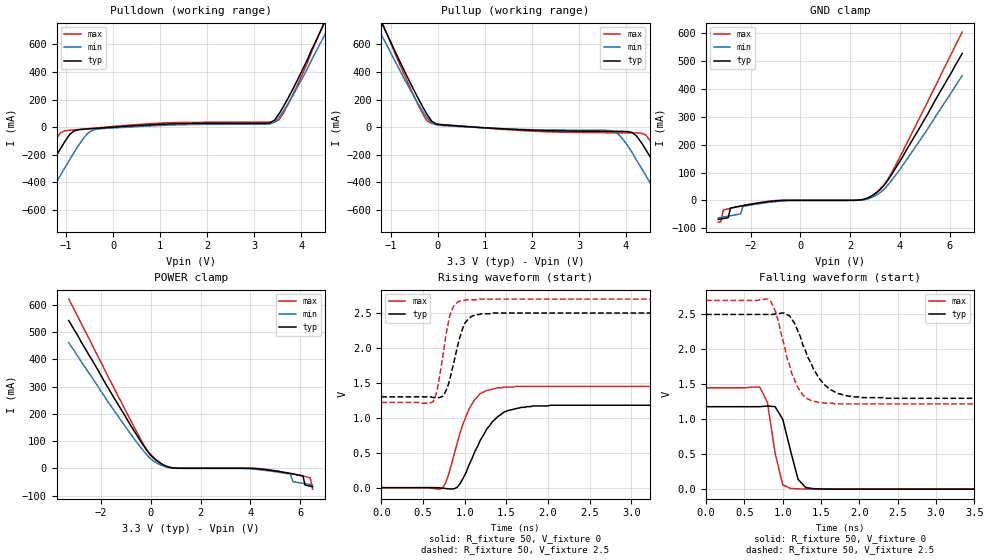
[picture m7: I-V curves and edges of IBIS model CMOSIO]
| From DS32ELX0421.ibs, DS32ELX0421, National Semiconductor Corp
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|   Model CMOSIO
[Model]  CMOSIO
Model_type I/O
Enable   Active-High
Vinl =   0
Vinh =   2
Vmeas =  1
C_comp   71.84fF   68.08fF   75.60fF
[Temperature Range]   25.0000   85.0000   -40.0000
[Voltage Range]   3.3000V   3.0000V   3.4650V
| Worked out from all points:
|   slope of the pulldown table from 0 to 0.495 V, typ, clamps not added: 44.3 ohm
|   slope of the pullup table from 0 to 0.495 V, typ, clamps not added: 36.2 ohm
|   GND clamp passes 1 mA (typ) near -0.87 V on its own axis
|   rising waveform, R_fixture 50, V_fixture 0: 20-80 % time 310ps typ, NA min, 238ps max; typ from 0 V to 1.18 V
|   rising waveform, R_fixture 50, V_fixture 2.5: 20-80 % time 151ps typ, NA min, 123ps max; typ from 1.3 V to 2.5 V
|   falling waveform, R_fixture 50, V_fixture 0: 20-80 % time 164ps typ, NA min, 139ps max; typ from 1.18 V to 0 V
|   falling waveform, R_fixture 50, V_fixture 2.5: 20-80 % time 312ps typ, NA min, 231ps max; typ from 2.5 V to 1.3 V
[GND_clamp]
|Voltage   I(typ)   I(min)   I(max)
-3.3V     -68.7mA    -62.7mA    -78.5mA
-3.2V     -67.1mA    -61.3mA    -76.7mA
-3.1V     -65.4mA    -59.8mA    -34.7mA
-2.9V     -62mA      -56.8mA    -30.4mA
-2.81V    -27.9mA    -55.3mA    -28.4mA
-2.41V    -20.8mA    -49.1mA    -20.8mA
-2.31V    -19.1mA    -21.5mA    -19mA
-1.82V    -11.5mA    -14.1mA    -10.5mA
2.44V     2.08mA     1.33mA     986uA
2.94V     20.3mA     13.6mA     19.9mA
3.73V     102mA      79.3mA     110mA
6.5V      528mA      448mA      605mA
|6.60E+00   5.43E-01   4.62E-01   6.22E-01
[POWER_clamp]
|Voltage   I(typ)   I(min)   I(max)
|6.60E+00   -6.87E-02   -6.27E-02   -7.85E-02
-3.3V     543mA      462mA      622mA
-330mV    88.4mA     67.9mA     93.6mA
363mV     20.3mA     13.6mA     19.9mA
858mV     2.08mA     1.33mA     986uA
3.73V     -712nA     -332uA     -928pA
5.12V     -11.5mA    -14.1mA    -10.5mA
5.61V     -19.1mA    -21.5mA    -19mA
5.71V     -20.8mA    -49.1mA    -20.8mA
6.11V     -27.9mA    -55.3mA    -28.4mA
6.2V      -62mA      -56.8mA    -30.4mA
6.4V      -65.4mA    -59.8mA    -34.7mA
6.5V      -67.1mA    -61.3mA    -76.7mA
[Pulldown]
|Voltage   I(typ)   I(min)   I(max)
-3.3V     -1.59A     -1.67A     -1.61A
-2.21V    -858mA     -1A        -788mA
-2.01V    -726mA     -883mA     -640mA
-1.72V    -530mA     -703mA     -424mA
-1.22V    -216mA     -408mA     -89.8mA
-1.02V    -102mA     -293mA     -26.7mA
-627mV    -15.2mA    -80.9mA    -14mA
-330mV    -8.06mA    -13.8mA    -5.07mA
3.43V     50.2mA     35.9mA     37.2mA
3.63V     154mA      121mA      107mA
4.52V     775mA      682mA      785mA
6.5V      2.23A      2.01A      2.41A
|6.60E+00   2.30E+00   2.08E+00   2.49E+00
[Pullup]
|Voltage   I(typ)   I(min)   I(max)
|6.60E+00   -1.59E+00   -1.67E+00   -1.61E+00
-3.3V     2.3A       2.08A      2.49A
-1.22V    775mA      682mA      785mA
-1.12V    703mA      617mA      705mA
-330mV    153mA      120mA      101mA
-132mV    44.3mA     30.8mA     26.6mA
3.73V     -30.5mA    -30.3mA    -40.8mA
4.13V     -38.6mA    -184mA     -41.7mA
4.42V     -163mA     -350mA     -56.7mA
5.02V     -530mA     -703mA     -426mA
5.31V     -726mA     -883mA     -640mA
5.41V     -792mA     -943mA     -714mA
6.5V      -1.52A     -1.61A     -1.53A
[Ramp]
|variable   typ   min   max
dV/dt_r   156.00m/266.4p   155.98m/289.5p   155.97m/245.7p
dV/dt_f   156.025m/256.2p  156.016m/278.8p   155.988m/237.1p
R_load  = 50
[Rising Waveform]
R_fixture=   50
V_fixture=   0
V_fixture_min=  0
V_fixture_max=  0
|time   V(typ)   V(min)   V(max)
0s        683pV      NA         627pV
735ps     -7.06mV    NA         -3.5mV
805ps     -16.2mV    NA         178mV
910ps     5.69mV     NA         634mV
1.05ns    320mV      NA         1.12V
1.19ns    685mV      NA         1.35V
1.4ns     1.02V      NA         1.43V
1.68ns    1.15V      NA         1.45V
2.03ns    1.18V      NA         1.45V
10ns      1.18V      NA         1.45V
[Rising Waveform]
R_fixture=   50
V_fixture=   2.5
V_fixture_min=  2.3
V_fixture_max=  2.7
|time   V(typ)   V(min)   V(max)
0s        1.3V       NA         1.22V
620ps     1.29V      NA         1.23V
680ps     1.29V      NA         1.46V
740ps     1.31V      NA         1.9V
820ps     1.54V      NA         2.45V
880ps     1.84V      NA         2.62V
960ps     2.22V      NA         2.67V
1.02ns    2.38V      NA         2.69V
1.34ns    2.5V       NA         2.7V
10ns      2.5V       NA         2.7V
[Falling Waveform]
R_fixture=   50
V_fixture=   0
V_fixture_min=  0
V_fixture_max=  0
|time   V(typ)   V(min)   V(max)
0s        1.18V      NA         1.45V
700ps     1.18V      NA         1.46V
800ps     1.19V      NA         1.24V
900ps     1.18V      NA         517mV
1ns       1V         NA         61.9mV
1.1ns     556mV      NA         11mV
1.2ns     140mV      NA         4.73mV
1.3ns     23.7mV     NA         3.08mV
1.4ns     6.86mV     NA         2.63mV
10ns      559nV      NA         420nV
[Falling Waveform]
R_fixture=   50
V_fixture=   2.5
V_fixture_min=  2.3
V_fixture_max=  2.7
|time   V(typ)   V(min)   V(max)
0s        2.5V       NA         2.7V
840ps     2.5V       NA         2.69V
910ps     2.51V      NA         2.53V
1.09ns    2.48V      NA         1.77V
1.19ns    2.28V      NA         1.47V
1.3ns     1.97V      NA         1.31V
1.47ns    1.59V      NA         1.24V
1.68ns    1.39V      NA         1.22V
2.03ns    1.31V      NA         1.22V
10ns      1.3V       NA         1.22V
